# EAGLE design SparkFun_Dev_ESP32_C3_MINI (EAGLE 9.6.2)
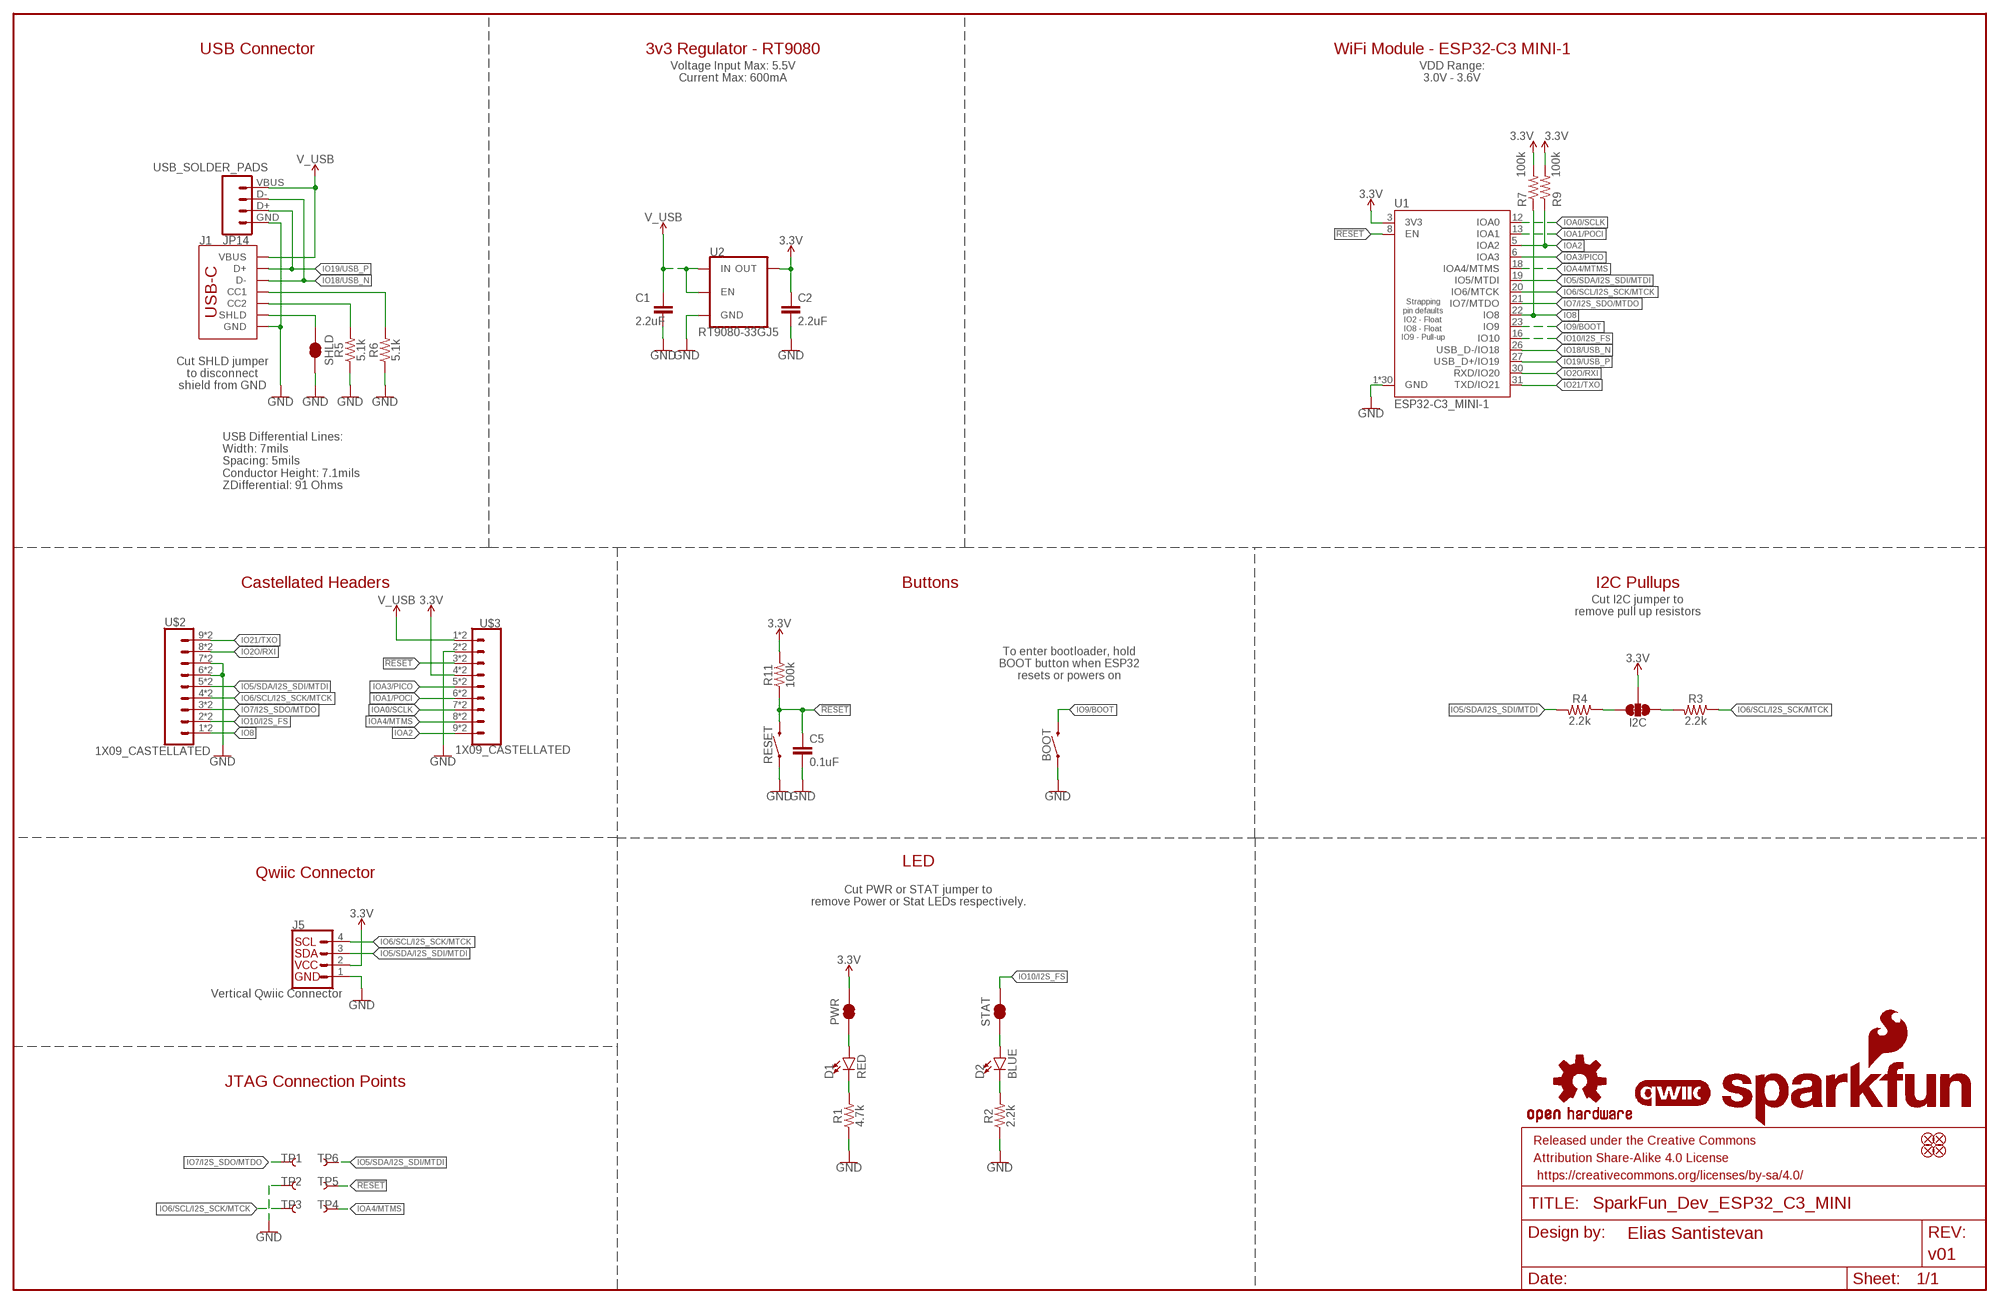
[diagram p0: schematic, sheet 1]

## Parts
BOOT  MOMENTARY-SWITCH-SPST-SMD-4.6X2.8MM  [TACTILE_SWITCH_SMD_4.6X2.8MM]
C1  2.2uF  2.2UF-0402_TIGHT-10V-10%-X5R  [0402-TIGHT]
C2  2.2uF  2.2UF-0402_TIGHT-10V-10%-X5R  [0402-TIGHT]
C5  0.1uF  0.1UF-0402T-6.3V-10%-X7R  [0402-TIGHT]
D1  RED  LED-RED_0603-KB  [LED-0603]
D2  BLUE  LED-BLUE0603  [LED-0603]
FD1  FIDUCIALUFIDUCIAL  [FIDUCIAL-MICRO]
FD2  FIDUCIALUFIDUCIAL  [FIDUCIAL-MICRO]
FD3  FIDUCIALUFIDUCIAL  [FIDUCIAL-MICRO]
FD4  FIDUCIALUFIDUCIAL  [FIDUCIAL-MICRO]
FRAME2  FRAME-LEDGER  [CREATIVE_COMMONS]
I2C  JUMPER-SMT_3_2-NC_TRACE_SILK  [SMT-JUMPER_3_2-NC_TRACE_SILK]
J1  USB Female Type C Connector  USB_C_4-LAYER_PADS  [USB-C-16P_4LAYER-PADS]
J5  Vertical Qwiic Connector  QWIIC_CONNECTOR  [JST04_1MM_VERT]
JP14  USB_SOLDER_PADS  [USB-SOLDER-PADS]
LOGO1  SFE_LOGO_NAME_FLAMEBLANK  [BLANK]
LOGO2  QWIIC_LOGO_3MM  [QWIIC_3MM]
LOGO3  OSHW-LOGOS  [OSHW-LOGO-S]
PWR  JUMPER-SMT_2_NC_TRACE_SILK  [SMT-JUMPER_2_NC_TRACE_SILK]
R1  4.7k  4.7KOHM-0402T-1/16W-1%  [0402-TIGHT]
R2  2.2k  2.2KOHM-0402T-1/16W-1%  [0402-TIGHT]
R3  2.2k  2.2KOHM-0402T-1/16W-1%  [0402-TIGHT]
R4  2.2k  2.2KOHM-0402T-1/16W-1%  [0402-TIGHT]
R5  5.1k  5.1KOHM-0402T-1/16W-1%  [0402-TIGHT]
R6  5.1k  5.1KOHM-0402T-1/16W-1%  [0402-TIGHT]
R7  100k  100KOHM-0402T-1/16W-1%  [0402-TIGHT]
R9  100k  100KOHM-0402T-1/16W-1%  [0402-TIGHT]
R11  100k  100KOHM-0402T-1/16W-1%  [0402-TIGHT]
RESET  MOMENTARY-SWITCH-SPST-SMD-4.6X2.8MM  [TACTILE_SWITCH_SMD_4.6X2.8MM]
SHLD  JUMPER-SMT_2_NC_TRACE_SILK  [SMT-JUMPER_2_NC_TRACE_SILK]
STAT  JUMPER-SMT_2_NC_TRACE_SILK  [SMT-JUMPER_2_NC_TRACE_SILK]
TP1  TEST-POINT3X5  [PAD.03X.05]
TP2  TEST-POINT3X5  [PAD.03X.05]
TP3  TEST-POINT3X5  [PAD.03X.05]
TP4  TEST-POINT3X5  [PAD.03X.05]
TP5  TEST-POINT3X5  [PAD.03X.05]
TP6  TEST-POINT3X5  [PAD.03X.05]
U1  ESP32-C3_MINI-1  [ESP32-C3-MINI-1]
U2  RT9080-33GJ5  V_REG_RT9080  [SOT23-5]
U$2  1X09_CASTELLATED  [1X09_CASTELLATED]
U$3  1X09_CASTELLATED  [1X09_CASTELLATED]

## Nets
3.3V: C2.1 I2C.2 J5.2 PWR.2 R7.2 R9.2 R11.2 U1.3(3V3) U2.5(OUT) U$3.4 U$3.4B
!RESET!: C5.1 R11.1 RESET.3 RESET.4 TP5.1 U1.8(EN) U$3.3 U$3.3B
GND: BOOT.1 BOOT.2 C1.2 C2.2 C5.2 J1.GND J1.GND2(GND) J5.1 JP14.GND R1.1 R2.1 R5.1 R6.1 RESET.1 RESET.2 SHLD.2 TP2.1 U1.1(GND) U1.2(GND) U1.11(GND) U1.14(GND) U1.36(GND) U1.37(GND) U1.38(GND) U1.39(GND) U1.40(GND) U1.41(GND) U1.42(GND) U1.43(GND) U1.44(GND) U1.45(GND) U1.46(GND) U1.47(GND) U1.48(GND) U1.49.1(GND) U1.49.2(GND) U1.49.3(GND) U1.49.4(GND) U1.49.5(GND) U1.49.6(GND) U1.49.7(GND) U1.49.8(GND) U1.49.9(GND) U1.50(GND) U1.51(GND) U1.52(GND) U1.53(GND) U2.2(GND) U$2.6 U$2.6B U$2.7 U$2.7B U$3.2 U$3.2B
IO2O/RXI: U1.30(RXD/IO20) U$2.8 U$2.8B
IO5/SDA/I2S_SDI/MTDI: J5.3 R4.2 TP6.1 U1.19(IO5/MTDI) U$2.5 U$2.5B
IO6/SCL/I2S_SCK/MTCK: J5.4 R3.1 TP3.1 U1.20(IO6/MTCK) U$2.4 U$2.4B
IO7/I2S_SDO/MTDO: TP1.1 U1.21(IO7/MTDO) U$2.3 U$2.3B
IO8: R7.1 U1.22(IO8) U$2.1 U$2.1B
IO9/BOOT: BOOT.3 BOOT.4 U1.23(IO9)
IO10/I2S_FS: STAT.2 U1.16(IO10) U$2.2 U$2.2B
IO18/USB_N [USB]: J1.A7(D-) J1.B7(D-) JP14.D- U1.26(USB_D-/IO18)
IO19/USB_P [USB]: J1.A6(D+) J1.B6(D+) JP14.D+ U1.27(USB_D+/IO19)
IO21/TXO: U1.31(TXD/IO21) U$2.9 U$2.9B
IOA0/SCLK: U1.12(IOA0) U$3.7 U$3.7B
IOA1/POCI: U1.13(IOA1) U$3.6 U$3.6B
IOA2: R9.1 U1.5(IOA2) U$3.9 U$3.9B
IOA3/PICO: U1.6(IOA3) U$3.5 U$3.5B
IOA4/MTMS: TP4.1 U1.18(IOA4/MTMS) U$3.8 U$3.8B
N$1: D1.C R1.2
N$2: D1.A PWR.1
N$3: D2.C R2.2
N$4: I2C.3 R3.2
N$5: I2C.1 R4.1
N$7: J1.B5(CC2) R5.2
N$8: J1.A5(CC1) R6.2
N$11: D2.A STAT.1
SHLD: J1.SHLD1(SHLD) J1.SHLD2(SHLD) J1.SHLD3(SHLD) J1.SHLD4(SHLD) SHLD.1
V_USB: C1.1 J1.VBUS1(VBUS) J1.VBUS2(VBUS) JP14.VBUS U2.1(IN) U2.3(EN) U$3.1 U$3.1B

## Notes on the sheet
- USB Connector | 3v3 Regulator - RT9080 | WiFi Module - ESP32-C3 MINI-1
- Voltage Input Max: 5.5V
  Current Max: 600mA
- VDD Range:
  3.0V - 3.6V
- Cut SHLD jumper
  to disconnect
  shield from GND
- USB Differential Lines:  
  Width: 7mils
  Spacing: 5mils
  Conductor Height: 7.1mils
  ZDifferential: 91 Ohms
- Castellated Headers | Buttons | I2C Pullups
- Cut I2C jumper to
  remove pull up resistors
- To enter bootloader, hold
  BOOT button when ESP32
  resets or powers on
- LED
- Qwiic Connector
- Cut PWR or STAT jumper to
  remove Power or Stat LEDs respectively.
- JTAG Connection Points

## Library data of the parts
BOOT RESET = SparkFun-Switches:MOMENTARY-SWITCH-SPST: Momentary Switch (Pushbutton) - SPST; PROD_ID: SWCH-15606
C1 C2 = SparkFun-Capacitors:2.2UF: 2.2µF ceramic capacitors; PROD_ID: CAP-14232
C5 = SparkFun-Capacitors:0.1UF: 0.1µF ceramic capacitors; PROD_ID: CAP-14993
D1 = SparkFun-LED:LED-RED: Red SMD LED; PROD_ID: DIO-17976
D2 = SparkFun-LED:LED-BLUE: Blue SMD LED; PROD_ID: DIO-08575
FD1-FD4 = SparkFun-Aesthetics:FIDUCIAL: Fiducial Alignment Points
FRAME2 = SparkFun-Aesthetics:FRAME-LEDGER: Schematic Frame - Ledger; DESIGNER: Elias Santistevan; REV: v01
I2C = SparkFun-Jumpers:JUMPER-SMT_3_2-NC_TRACE: Normally closed trace jumper (2 of 2 connections) This jumper has a trace between all three pads so they are normally closed (NC). Use a razor knife to open the connection(s). For best results follow the IPC guidelines for cutting traces: Cutout at least 0.063 mm (0.005 in). Remove all loose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
J1 = SparkFun-Connectors:USB_C: USB Type C 16Pin Connector Super Speed pins not available on the 16-pin purely SMD connector so this part is best for USB 2.0 implementations. D1 and D2 are tied together enabling D+/- no matter which way the cable is plugged into the connector. The two channel configuration pins (CC1/2) are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; PROD_ID: CONN-14122
J5 = SparkFun-Connectors:QWIIC_CONNECTOR: SparkFun I2C Standard Qwiic Connector An SMD 1mm pitch JST connector makes it easy and quick (get it? Qwiic?) to connect I2C devices to each other. The Qwiic system enables fast and solderless connection between popular platforms and various sensors and actuators. We carry 200mm, 100mm, 50mm, and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; PROD_ID: CONN-14483
JP14 = SparkFun-Connectors:USB_SOLDER_PADS: Solder pad access to USB pins. Helpful to expose on PCBs so user can attach external USB connector if necessary.
LOGO1 = SparkFun-Aesthetics:SFE_LOGO_NAME_FLAME: SparkFun Font Logo w/ Flame
LOGO2 = SparkFun-Aesthetics:QWIIC_LOGO: Qwiic Logos for placement on schematic and PCB. The 5.5mm silk logo is best for placing next to Qwiic connector.
LOGO3 = SparkFun-Aesthetics:OSHW-LOGO: Open-Source Hardware (OSHW) Logo
PWR SHLD STAT = SparkFun-Jumpers:JUMPER-SMT_2_NC_TRACE: Normally closed trace jumper
R1 = SparkFun-Resistors:4.7KOHM: 4.7kΩ resistor; PROD_ID: RES-15343
R2-R4 = SparkFun-Resistors:2.2KOHM: 2.2kΩ resistor; PROD_ID: RES-14341
R5 R6 = SparkFun-Resistors:5.1KOHM; PROD_ID: RES-14340
R7 R9 R11 = SparkFun-Resistors:100KOHM: 100kΩ resistor; PROD_ID: RES-13495
TP1-TP6 = SparkFun-Connectors:TEST-POINT: SparkFun Test Points
U1 = ESP32-C3-MINI-1:ESP32-C3_MINI-1: Espressif ESP32C3-MINI-1 ESP32-C3-MINI-1 and ESP32-C3-MINI-1U are two general-purpose Wi-Fi and Bluetooth LE modules. The rich set of peripherals and a small size make the two modules an ideal choice for smart homes, industrial automation, health care, consumer electronics, etc. ESP32-C3-MINI-1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; PROD_ID: IC-20056
U2 = SparkFun-IC-Power:V_REG_RT9080; PROD_ID: VREG-19034
U$2 U$3 = ESP32-C3-MINI-1:1X09_CASTELLATED

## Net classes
1 Power: width 0.127 mm, clearance 0.178 mm
2 USB: width 0.178 mm, clearance 0.127 mm

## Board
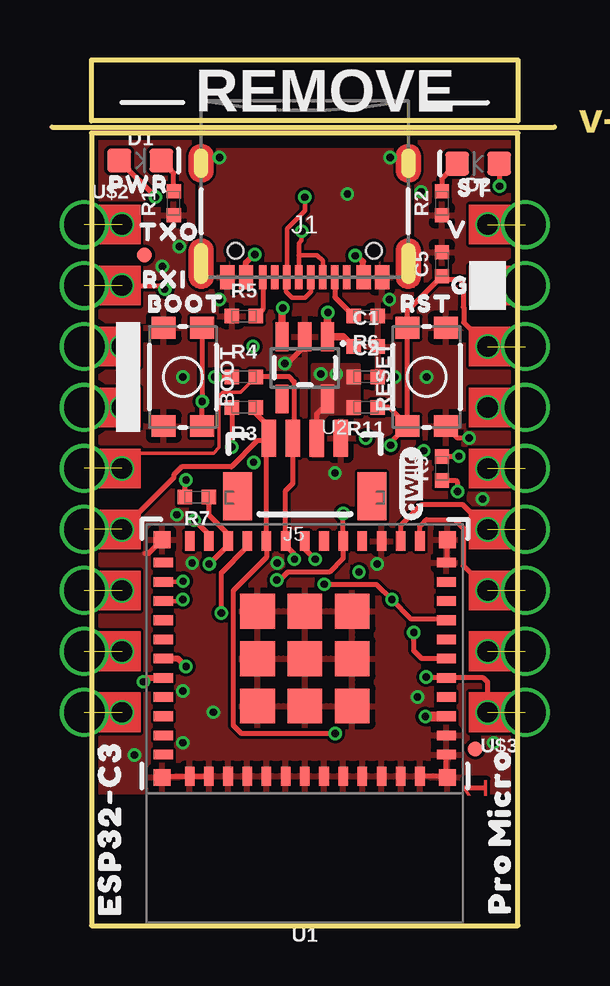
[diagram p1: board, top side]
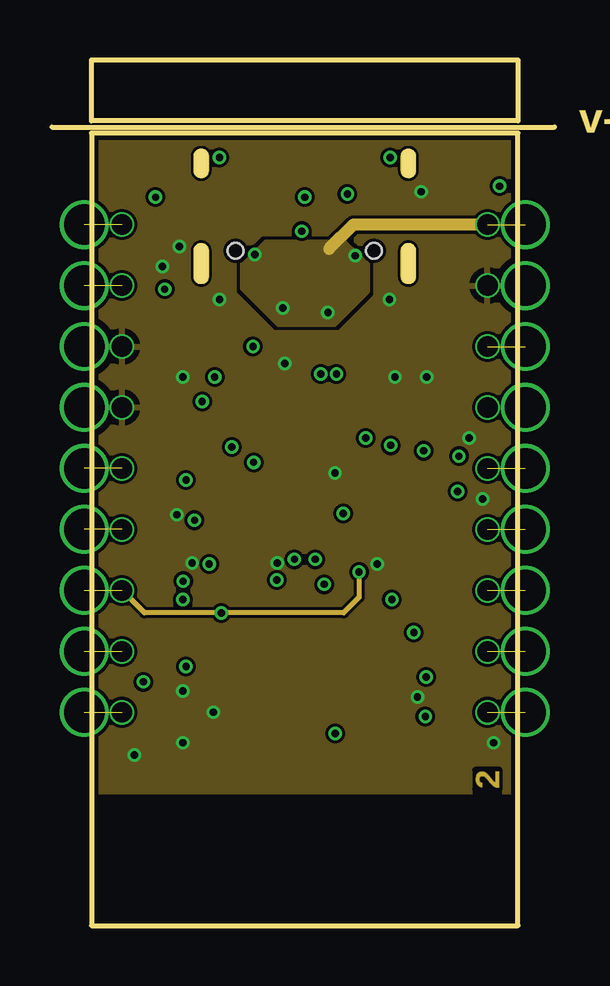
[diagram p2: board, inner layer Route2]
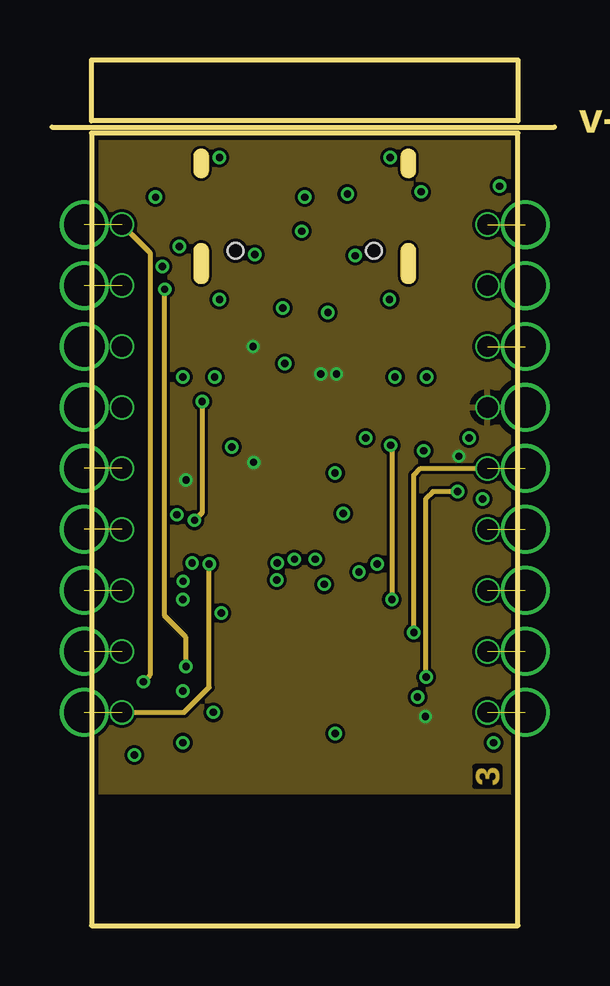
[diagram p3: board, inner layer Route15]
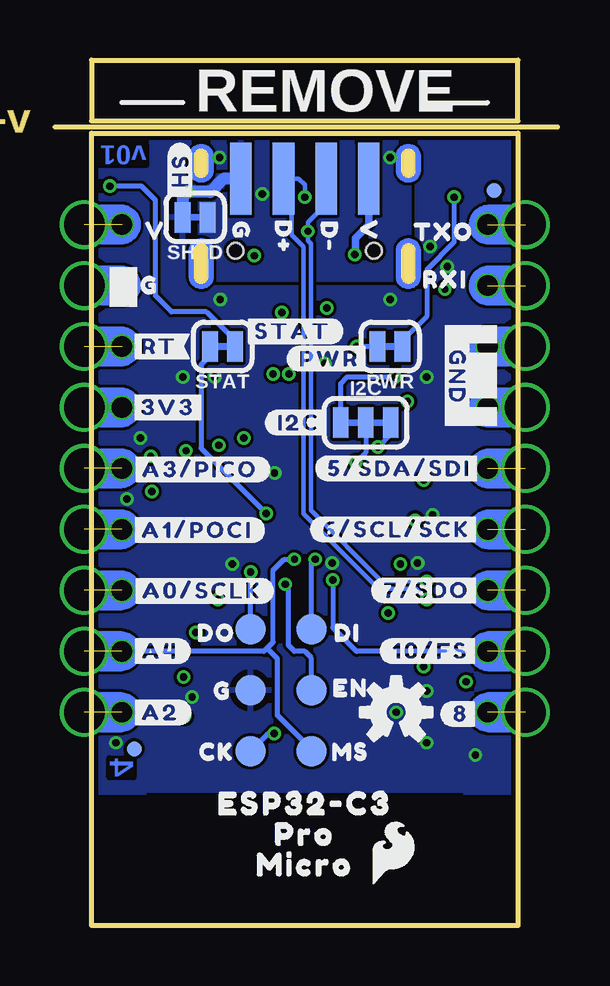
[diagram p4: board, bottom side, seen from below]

Size 17.78 x 36.07 mm. Coordinates in mm from the lower left corner, seen from the top.
Outline: 0,33.02 0,0 17.78,0 17.78,33.02 0,33.02
Outline: 17.78,33.53 0,33.53 0,36.07 17.78,36.07 17.78,33.53
Copper layers (1*2*15*16): Top 0.035559375mm / dielectric 0.47751875mm / Route2 0.035559375mm / dielectric 0.47751875mm / Route15 0.035559375mm / dielectric 0.47751875mm / Bottom 0.035559375mm
Design rules "SparkFun-4-Layer-Minimum-JLCPCB *": minimum track width 5mil, minimum drill 0.2mm, track to track 5mil, track to pad 5mil, pad to pad 5mil, via to via 5mil, smd to smd 5mil, copper to edge 7mil, drill to drill 7mil, minimum pad ring 3mil, minimum via ring 5mil, stop-mask expansion 2.5mil, vias tented up to drill 25mil, thermal gap 10mil
Milling: 1 lines

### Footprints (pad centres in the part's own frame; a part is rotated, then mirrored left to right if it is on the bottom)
TACTILE_SWITCH_SMD_4.6X2.8MM = smd 0.9 x 1: 1 -2.05,-0.8; 2 2.05,-0.8; 3 2.05,0.8; 4 -2.05,0.8
0402-TIGHT = smd 0.6 x 0.6: 1 -0.5,0; 2 0.5,0
LED-0603 = smd 1 x 1: A -0.877,0; C 0.877,0
FIDUCIAL-MICRO = smd 0.635 x 0.635: 1 0,0
SMT-JUMPER_3_2-NC_TRACE_SILK = smd 0.66 x 1.27: 1 -1.041,0; 2 0,0; 3 1.041,0
USB-C-16P_4LAYER-PADS = smd 0.3 x 1: A5 -1.25,-0.34; A6 -0.25,-0.34; A7 0.25,-0.34; A8 1.25,-0.34; B5 1.75,-0.34; B6 0.75,-0.34; B7 -0.75,-0.34; B8 -1.75,-0.34 | smd 0.6 x 1: GND -3.225,-0.34; GND2 3.225,-0.34; VBUS1 -2.45,-0.34; VBUS2 2.45,-0.34 | drill 0.4 pad 0.6 long: SHLD1 -4.318,-0.915; SHLD2 4.318,-0.915; SHLD3 -4.318,-5.095; SHLD4 4.318,-5.095 | hole 0.65: -2.89,-1.445; 2.89,-1.445
JST04_1MM_VERT = smd 0.6 x 1.55: 1 -1.5,0.775; 2 -0.5,0.775; 3 0.5,0.775; 4 1.5,0.775 | smd 1.2 x 2: NC1 -2.8,3.2; NC2 2.8,3.2
USB-SOLDER-PADS = smd 3 x 0.9: D+ 0,-0.889; D- 0,0.889; GND 0,-2.667; VBUS 0,2.667
SMT-JUMPER_2_NC_TRACE_SILK = smd 0.66 x 1.27: 1 -0.521,0; 2 0.521,0
PAD.03X.05 = smd 1.27 x 1.27: 1 0,0
ESP32-C3-MINI-1 = smd 0.8 x 0.4: 1 -5.9,4; 2 -5.9,3.2; 3 -5.9,2.4; 4 -5.9,1.6; 5 -5.9,0.8; 6 -5.9,0; 7 -5.9,-0.8; 8 -5.9,-1.6; 9 -5.9,-2.4; 10 -5.9,-3.2; 11 -5.9,-4; 25 5.9,-4; 26 5.9,-3.2; 27 5.9,-2.4; 28 5.9,-1.6; 29 5.9,-0.8; 30 5.9,0; 31 5.9,0.8; 32 5.9,1.6; 33 5.9,2.4; 34 5.9,3.2; 35 5.9,4 | smd 0.4 x 0.8: 12 -4.8,-4.9; 13 -4,-4.9; 14 -3.2,-4.9; 15 -2.4,-4.9; 16 -1.6,-4.9; 17 -0.8,-4.9; 18 0,-4.9; 19 0.8,-4.9; 20 1.6,-4.9; 21 2.4,-4.9; 22 3.2,-4.9; 23 4,-4.9; 24 4.8,-4.9; 36 4.8,4.9; 37 4,4.9; 38 3.2,4.9; 39 2.4,4.9; 40 1.6,4.9; 41 0.8,4.9; 42 0,4.9; 43 -0.8,4.9; 44 -1.6,4.9; 45 -2.4,4.9; 46 -3.2,4.9; 47 -4,4.9; 48 -4.8,4.9 | smd 1.45 x 1.45: 49.1 -1.975,1.975; 49.2 -1.975,0; 49.3 -1.975,-1.975; 49.4 0,-1.975; 49.5 1.975,-1.975; 49.6 1.975,0; 49.7 1.975,1.975; 49.8 0,1.975; 49.9 0,0 | smd 0.7 x 0.7: 50 5.95,4.95; 51 5.95,-4.95; 52 -5.95,-4.95; 53 -5.95,4.95
SOT23-5 = smd 0.55 x 1.2: 1 -0.95,-1.3; 2 0,-1.3; 3 0.95,-1.3; 4 0.95,1.3; 5 -0.95,1.3
1X09_CASTELLATED = drill 0.85 pad 1.016: 1 0,0; 2 0,2.54; 3 0,5.08; 4 0,7.62; 5 0,10.16; 6 0,12.7; 7 0,15.24; 8 0,17.78; 9 0,20.32 | drill 1.7 pad 1.75: 1B -1.57,0; 2B -1.57,2.54; 3B -1.57,5.08; 4B -1.57,7.62; 5B -1.57,10.16; 6B -1.57,12.7; 7B -1.57,15.24; 8B -1.57,17.78; 9B -1.57,20.32

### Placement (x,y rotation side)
BOOT  3.81,22.86 270 top
C1  11.43,24.13 0 top
C2  11.43,22.86 0 top
C5  14.61,27.56 90 top
D1  2.03,31.88 0 top
D2  16.12,31.75 180 top
FD1  0.99,30.63 0 bottom
FD2  2.21,27.94 0 top
FD3  16,7.37 0 top
FD4  16,7.37 0 bottom
FRAME2  not placed on the board
I2C  6.35,20.95 0 bottom
J1  8.89,26.67 180 top
J5  8.89,21.08 180 top
JP14  8.89,31.11 270 bottom
LOGO1  not placed on the board
LOGO2  13.34,18.41 90 top
LOGO3  5.08,8.89 0 bottom
PWR  5.33,24.13 180 bottom
R1  3.43,30.1 90 top
R2  14.61,30.1 90 top
R3  6.35,21.59 180 top
R4  6.35,22.86 0 top
R5  6.35,25.4 0 top
R6  11.43,25.4 180 top
R7  4.39,17.86 180 top
R9  14.61,19.05 90 top
R11  11.43,21.59 180 top
RESET  13.97,22.86 90 top
SHLD  13.46,29.51 180 bottom
STAT  12.32,24.13 180 bottom
TP1  11.16,12.34 0 bottom
TP2  11.16,9.8 0 bottom
TP3  11.16,7.26 0 bottom
TP4  8.62,7.26 0 bottom
TP5  8.62,9.8 0 bottom
TP6  8.62,12.34 0 bottom
U1  8.89,11.13 180 top
U2  8.89,23.24 180 top
U$1  [G36]  15.37,26.67 0 bottom
U$2  1.27,8.89 0 top
U$3  16.51,29.21 180 top
U$4  [#GND#4]  2.54,22.86 270 bottom
U$5  [RST41]  13.97,25.91 0 top
U$6  [#I2C#43]  9.14,20.95 0 bottom
U$7  [#PWR#47]  7.87,23.62 0 bottom
U$8  [#STAT#48]  9.4,24.77 0 bottom
U$9  [#SH#44]  14.1,31.37 270 bottom
U$10  [TXO40]  3.1,28.91 0 bottom
U$11  [RXI39]  3.05,26.92 0 bottom
U$12  [#3V3#0]  14.61,21.59 0 bottom
U$13  [#A3#PICO#35]  13.27,19.01 0 bottom
U$14  [#A1#POCI#35]  13.39,16.48 0 bottom
U$15  [#A2#35]  14.92,8.88 0 bottom
U$16  [#A0#SCLK#35]  13.19,13.95 0 bottom
U$17  [#A4#35]  14.93,11.44 0 bottom
U$18  [#8#35]  2.39,8.82 0 bottom
U$19  [#10#FS#35]  3.65,11.44 0 bottom
U$20  [#5#SDA#SDI#49]  4.95,19.05 0 bottom
U$21  [#6#SCL#SCK#49]  5.08,16.51 0 bottom
U$22  [#7#SDO#49]  3.81,13.97 0 bottom
U$23  [CK39]  12.57,7.24 0 bottom
U$24  [ORDERING_INSTRUCTIONS]  not placed on the board
U$25  [D#33]  9.78,28.7 270 bottom
U$26  [D#34]  7.87,28.7 270 bottom
U$27  [DI36]  7.11,12.19 0 bottom
U$28  [DO35]  12.57,12.19 0 bottom
U$29  [EN37]  6.99,9.91 0 bottom
U$30  [MS38]  6.99,7.24 0 bottom
U$31  [G36]  11.56,28.96 270 bottom
U$32  [V35]  6.22,28.96 270 bottom
U$33  [G36]  12.32,9.78 0 bottom
U$34  [ESP32#C32]  8.89,5.08 0 bottom
U$35  [PRO0]  8.89,3.81 0 bottom
U$36  [MICRO1]  8.89,2.54 0 bottom
U$37  [V35]  15.11,28.96 0 bottom
U$38  [V35]  15.27,29.01 0 top
U$39  [G36]  15.37,26.67 0 top
U$41  [BOOT15]  3.94,25.91 0 top
U$42  [RXI39]  3.05,26.92 0 top
U$43  [TXO40]  3.25,28.91 0 top
U$44  [PWR17]  1.96,30.89 0 top
U$45  [ESP32#C32]  0.76,4.06 90 top
U$46  [PRO0]  17.02,1.78 90 top
U$47  [MICRO1]  17.02,5.33 90 top
U$48  [SFE_LOGO_FLAME_.1]  5.21,3.05 0 bottom
U$49  [ST18]  16,30.73 0 top
U$51  [#RT#45]  14.96,24.13 0 bottom

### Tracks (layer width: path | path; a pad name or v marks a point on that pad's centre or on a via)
3.3V  (via drill 0.3)
  Top 0.203: J5.2 9.39,21.32 9.81,21.74 | R9.2 15.31,19.55 v15.32,19.56 | v3.94,18.57 3.89,18.52 R7.2
  Top 0.305: 9.81,21.74 9.81,21.96 9.84,21.99 U2.5
  Top 0.406: v13.92,8.71 13.93,8.72 U1.3
  Bottom 0.203: I2C.2 6.35,19.71 v6.76,19.3 | PWR.2 v6.73,24.13
  other vias: 10.21,22.99 9.55,22.99
  pour Route15 (rank 4): 0,33.02 17.78,33.02 17.78,5.59 0,5.59
  pour Top (no thermals): 9.19,19.56 9.65,19.56 9.65,21.08 9.91,21.34 11.18,21.34 11.18,23.37 9.19,23.37
!RESET!  (via drill 0.3)  (1 unrouted)
  Top 0.203: R11.1 12.39,21.59 RESET.4 | RESET.4 RESET.3 13.17,25.62 C5.1 14.74,26.92 15.37,26.92 15.49,26.8 15.49,25.78 15.52,25.76 15.52,25.12 U$3.3 | v12.47,20.02 12.47,20.12 RESET.4 | U1.8 14.74,12.78 13.34,12.78 v12.52,13.59 11.89,14.22 v9.7,14.22
  Route15 0.203: v12.47,20.02 12.52,19.96 v12.52,13.59
  Bottom 0.203: v9.7,14.22 9.58,14.1 9.58,11.68 9.32,11.43 8.89,11.43 8.62,11.16 TP5.1
GND  (via drill 0.3)
  Top 0.2: 14.79,6.22 U1.1 | U1.53 14.79,6.22 | 14.79,6.22 U1.48 | U1.50 2.99,6.22 U1.37 | U1.11 14.84,15.18 U1.52 | U1.51 2.36,15.5 2.23,15.5
  Top 0.203: 8.89,24.21 8.89,24.16 8.15,23.42 | RESET.1 15.26,20.32 v15.75,20.32
  Top 0.254: U2.2 8.89,24.21
  Bottom 0.508: JP14.GND 12.29,31.11 12.83,30.58 v13.75,30.58 13.98,30.34 SHLD.2
  other vias: 8.05,23.42 3.56,17.12 3.81,22.86 13.97,22.86 3.81,7.62 1.78,7.11 3.66,28.3 12.65,22.86 10.15,18.86 5.33,26.09 12.42,26.09 2.95,27.46 16.76,7.62 11.91,15.06 3.81,9.78 5.08,8.89 7.75,15.11 13.59,9.53 16.31,17.78 4.19,15.11
  pour Top (rank 4): 0,33.02 17.78,33.02 17.78,5.59 0,5.59
  pour Bottom (rank 4): 0,33.02 17.78,33.02 17.78,5.59 0,5.59
  pour Route2 (rank 4): 0,33.02 17.78,33.02 17.78,5.59 0,5.59
IO2O/RXI  (via drill 0.3)  (1 unrouted)
  Top 0.203: U$2.8 2.9,26.67 v3.05,26.52
  Top 0.254: v3.94,10.79 3.61,11.12 U1.30
  Route15 0.203: v3.94,10.79 3.94,12.01 3.05,12.9 v3.05,26.52
IO5/SDA/I2S_SDI/MTDI  (via drill 0.3)  (1 unrouted)
  Top 0.152: R4.2 6.21,22.23 5.46,22.23 5.32,22.09 5.32,19.93 5.08,19.68 1.9,19.68
  Top 0.203: 6.9,22.91 R4.2 8.26,22.86 8.44,22.67 8.44,20.36 J5.3 8.39,18.42 8.09,18.12 U1.19 8.09,15.85 8.46,15.48 v8.46,15.27 | 1.9,19.68 U$2.5
  Bottom 0.203: TP6.1 8.62,15.1 v8.46,15.27
IO6/SCL/I2S_SCK/MTCK  (via drill 0.3)  (1 unrouted)
  Top 0.203: J5.4 7.29,20.21 U1.20 7.29,15.34 5.92,13.97 5.92,8.33 6.25,8 v10.16,8 | J5.4 7.39,20.8 6.85,21.34 R3.1 | J5.4 7.28,20.19 6.91,20.19 5.83,19.11 3.76,19.11 3.43,18.78 3.43,18.67 U$2.4
  Bottom 0.203: TP3.1 10.41,8 v10.16,8
IO7/I2S_SDO/MTDO  (via drill 0.3)  (1 unrouted)
  Top 0.203: 6.49,15.76 U1.21 6.49,15.79 5.41,14.71 v5.41,13.03
  Route2 0.203: U$2.3 2.21,13.03 v5.41,13.03 10.51,13.03 11.15,13.67 v11.15,14.74
  Bottom 0.203: TP1.1 v11.16,14.73 v11.15,14.74
IO8  (via drill 0.3)  (1 unrouted)
  Top 0.203: 5.69,16.32 U1.22 | U1.22 5.69,16.3 4.89,17.09 R7.1 | U1.22 5.69,15.85 v4.9,15.06
  Route15 0.203: U$2.1 3.86,8.89 4.9,9.93 v4.9,15.06
IO9/BOOT  (via drill 0.3)
  Top 0.203: BOOT.4 v4.61,21.84 BOOT.3 | U1.23 4.89,16.29 v4.29,16.89
  Route15 0.203: v4.61,21.84 4.61,17.21 v4.29,16.89
IO10/I2S_FS  (via drill 0.3)  (1 unrouted)
  Top 0.203: v10.49,17.17 10.49,17.12 U1.16 10.49,15.3 9.92,14.73 8.18,14.73 7.85,14.4 v7.72,14.4
  Bottom 0.203: 12.42,24.13 STAT.2 12.84,23.75 13.22,23.37 13.22,19.9 v10.49,17.17 | U$2.2 6.73,11.43 7.72,12.42 v7.72,14.4
IO18/USB_N  (via drill 0.3)
  Top 0.178: J1.B7 9.64,27.7 9.4,27.94 8.64,27.94 J1.A7 8.64,28.43 8.76,28.55 v8.76,28.93 | v3.82,14.35 3.79,14.32 U1.26
  Bottom 0.178: JP14.D- 8,30.07 8.76,29.32 v8.76,28.93 8.76,28.54 8.64,28.42 8.64,17.3 5.69,14.35 v3.82,14.35
IO19/USB_P  (via drill 0.3)
  Top 0.178: J1.A6 9.14,26.41 8.89,26.16 8.35,26.16 8.11,26.41 8.11,26.98 J1.B6 8.14,29.04 8.89,29.79 v8.89,30.35 | U1.27 3.75,13.53 v3.81,13.59
  Bottom 0.178: v8.89,30.35 8.89,30.86 9.14,31.11 JP14.D+ 9.45,30.79 9.45,28.8 8.94,28.29 8.94,17.16 5.82,14.04 4.26,14.04 v3.81,13.59
IO21/TXO  (via drill 0.3)  (1 unrouted)
  Top 0.254: v2.16,10.16 2.32,10.32 U1.31
  Route15 0.203: U$2.9 2.44,28.04 2.44,10.44 v2.16,10.16
IOA0/SCLK  (1 unrouted)
  Top 0.203: U$3.7 15.49,14.99 15.49,16.56 15.14,16.92 13.97,16.92 13.77,16.71 13.69,16.64 U1.12
IOA1/POCI  (1 unrouted)
  Top 0.203: U1.13 12.89,16.68 13.77,17.55 15.47,17.55 U$3.6
IOA2  (via drill 0.3)  (1 unrouted)
  Top 0.203: U$3.9 16.51,10.16 16.34,10.32 U1.5 13.95,10.32 v13.95,10.36 | v15.27,18.09 15.27,18.47 15.18,18.55 R9.1
  Route15 0.203: v15.27,18.09 14.22,18.09 13.95,17.8 v13.95,10.36
IOA3/PICO  (via drill 0.3)  (1 unrouted)
  Top 0.203: U1.6 13.77,11.12 13.44,11.46 v13.44,12.22
  Route15 0.203: v13.44,12.22 13.44,18.77 13.72,19.05 U$3.5
IOA4/MTMS  (via drill 0.3)  (1 unrouted)
  Top 0.203: U1.18 8.88,16.02 8.88,15.71 v9.32,15.27
  Bottom 0.203: v9.32,15.27 9.75,15.27 10.21,14.81 10.21,11.81 10.46,11.56 | 10.46,11.56 10.59,11.43 U$3.8 | TP4.1 8.62,7.35 10.03,8.76 10.03,11.12 10.46,11.56
N$1
  Top 0.203: R1.2 3.43,31.36 D1.C
N$2  (via drill 0.3)
  Top 0.203: v2.67,30.35 2.67,30.36 D1.A
  Bottom 0.203: PWR.1 4.81,24.38 3.78,25.41 3.78,27.36 2.67,28.47 v2.67,30.35
N$3
  Top 0.203: R2.2 14.61,31.11 D2.C
N$4  (via drill 0.3)
  Top 0.203: R3.2 v5.85,19.95 v5.84,19.94
  Bottom 0.203: I2C.3 5.31,20.47 v5.84,19.94
N$5  (via drill 0.3)
  Top 0.203: R4.1 5.83,22.86 v5.13,22.86
  Bottom 0.203: I2C.1 7.39,22.58 7.11,22.86 v5.13,22.86
N$7
  Top 0.203: J1.B5 7.14,25.69 R5.2
N$8
  Top 0.203: J1.A5 10.14,26.19 R6.2
N$11  (via drill 0.3)
  Top 0.203: D2.A 16.99,30.83 v17.02,30.81
  Bottom 0.203: v17.02,30.81 15.7,30.81 15.11,30.23 15.11,26.24 14.45,25.58 12.99,25.58 11.8,24.38 STAT.1
N$13  (via drill 0.3)
  other vias: 13.84,19.79
N$16  (via drill 0.3)
  other vias: 11.43,20.32
SHLD  (via drill 0.3)
  other vias: 10.67,30.48 5.33,32 12.45,32
  pour Top (no thermals): 4.57,32.26 4.57,27.05 13.22,27.05 13.22,32.26
  pour Bottom (no thermals): 4.57,33.02 4.57,26.92 13.21,26.92 13.21,33.02
V_USB  (via drill 0.3)  (1 unrouted)
  Top 0.254: J1.VBUS1 11.32,27.03 11.32,27.67 11.08,27.91 v11,27.91 | J1.VBUS2 6.44,27.62 6.78,27.96 v6.81,27.96
  Top 0.305: v9.86,25.55 9.84,25.54 U2.1 10.47,24.54 10.89,24.13 C1.1 | U2.3 7.94,25.7 v7.98,25.73
  Route2 0.508: U$3.1 10.92,29.21 9.91,28.19
  Bottom 0.305: v6.81,27.96 6.78,27.99 6.78,28.64 6.22,29.2 JP14.VBUS
  pour Route2 (no thermals): 6.22,27.56 6.22,26.54 7.75,25.02 10.16,25.02 11.56,26.42 11.56,27.56 10.59,28.5 10.57,28.52 7.24,28.52 6.27,27.56

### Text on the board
Top: 1
Route2: 2
Route15: 3
Bottom: v01 | 4
tPlace: REMOVE
bPlace: REMOVE
Milling: v-score
Measures: Units: inches
tDocu: 4-layer / JLC7628 Stackup / Material: TG135-140 / 1oz outer layers / 0.5oz inner layers / Board thickness: 0.8mm / Soldermask: Red / Silkscreen: White / Surface Finish: Lead-Free HASL | Elias Santistevan

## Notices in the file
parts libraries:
SparkFun-Connectors: Licensing: Creative Commons ShareAlike 4.0 International - https://creativecommons.org/licenses/by-sa/4.0
SparkFun-Aesthetics: Released under the Creative Commons Attribution Share-Alike 4.0 License
SparkFun-Aesthetics: https://creativecommons.org/licenses/by-sa/4.0
